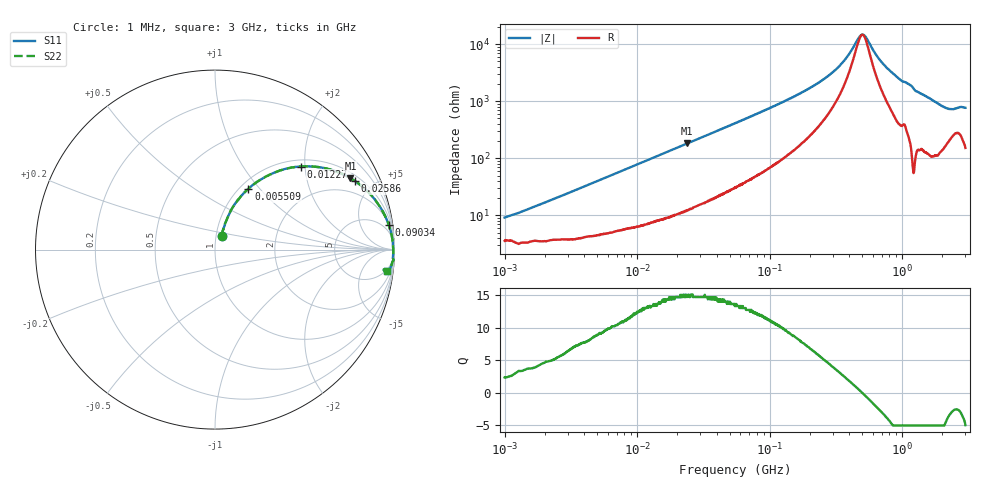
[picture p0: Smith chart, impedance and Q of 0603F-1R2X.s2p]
!s-Parameter Generated by FASTRON Sdn. Bhd.
!FASTRON P/N : 0603F-1R2X
!Keysight Technologies: E4991B_MY54100416_A.01.15
!Date: Wed Jun 19 15:42:30 2024
!Version  :Rev00  Wed Jun 19 15:42:30 2024
!Data & Calibration Information:
!Freq  S11  S21  S12  S22
!PortZ  Port1:50+j0  Port2:50+j0
!When reading reference impedance value at option line is always used.
! Remarks : This data is being provided solely for informational purposes.
# Hz S dB R 50
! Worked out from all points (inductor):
!   1601 points, 1 MHz to 3 GHz, reference 50 ohm
!   read as one part in series: L = 1.31 uH near 1.203 MHz
!   highest Q = 15 at 23.87 MHz (marker M1), where L = 1.21 uH
!   self-resonance near 500.5 MHz
!   S11 on the Smith chart (normalised r, x): 1 MHz: 1.07, +0.17; 5.509 MHz: 1.09, +0.87; 12.27 MHz: 1.14, +1.90; 25.86 MHz: 1.26, +3.93; 90.34 MHz: 2, +14; 3 GHz: 4, -15
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1000000  -21.10 62.3  -0.33 -4.6  -0.33 -4.6  -21.10 62.3
2065923  -15.70 68.9  -0.41 -9.2  -0.41 -9.2  -15.70 68.9
3804036  -11.00 66.2  -0.70 -16.3  -0.70 -16.3  -11.00 66.2
5508857  -8.26 61.2  -1.09 -22.6  -1.09 -22.6  -8.26 61.2
1.2268e7  -3.54 44.1  -3.12 -41.6  -3.12 -41.6  -3.54 44.1
1.447069e7  -2.85 39.9  -3.83 -45.9  -3.83 -45.9  -2.85 39.9
2.386763e7  -1.38 27.8  -6.60 -58.3  -6.60 -58.3  -1.38 27.8
2.585714e7  -1.22 26.1  -7.12 -60.1  -7.12 -60.1  -1.22 26.1
5.504702e7  -0.39 13.3  -12.70 -72.4  -12.70 -72.4  -0.39 13.3
9.034013e7  -0.20 8.2  -16.90 -76.9  -16.90 -76.9  -0.20 8.2
2.083556e8  -0.09 3.1  -25.20 -78.2  -25.20 -78.2  -0.09 3.1
3.285236e8  -0.07 1.4  -32.00 -71.7  -32.00 -71.7  -0.07 1.4
3.817355e8  -0.06 0.9  -35.50 -64.1  -35.50 -64.1  -0.06 0.9
4.686663e8  -0.06 0.2  -42.20 -28.0  -42.20 -28.0  -0.06 0.2
4.976708e8  -0.06 0.0  -43.40 -2.7  -43.40 -2.7  -0.06 0.0
5.311214e8  -0.06 -0.2  -42.60 26.3  -42.60 26.3  -0.06 -0.2
6.488164e8  -0.06 -0.9  -35.80 65.5  -35.80 65.5  -0.06 -0.9
7.925923e8  -0.06 -1.5  -31.20 75.0  -31.20 75.0  -0.06 -1.5
1.281378e9  -0.07 -3.8  -23.60 81.4  -23.60 81.4  -0.07 -3.8
2.040726e9  -0.25 -6.8  -18.40 72.8  -18.40 72.8  -0.25 -6.8
2.335937e9  -0.43 -7.2  -17.70 64.9  -17.70 64.9  -0.43 -7.2
3e9  -0.29 -7.1  -18.00 71.5  -18.00 71.5  -0.29 -7.1
